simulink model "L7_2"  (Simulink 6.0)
settings: Solver=ode3  StartTime=0.0  StopTime=10.0  RelTol=1e-3
libraries: simulink x1

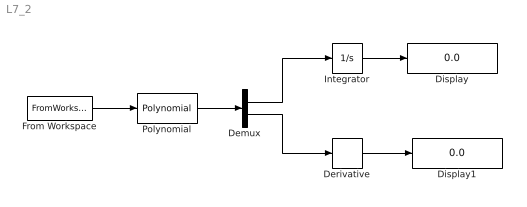
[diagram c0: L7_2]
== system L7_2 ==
  Demux : Demux  Outputs=2
  Derivative : Derivative
  Display : Display
  Display1 : Display
  From Workspace : FromWorkspace  VariableName=x  SampleTime=0
  Integrator : Integrator
  Polynomial : simulink/Math Operations/Polynomial  coefs=[1 2 4 1]
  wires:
  From Workspace/1 -> Polynomial/1
  Polynomial/1 -> Demux/1
  Demux/1 -> Integrator/1
  Integrator/1 -> Display/1
  Derivative/1 -> Display1/1
  Demux/2 -> Derivative/1
